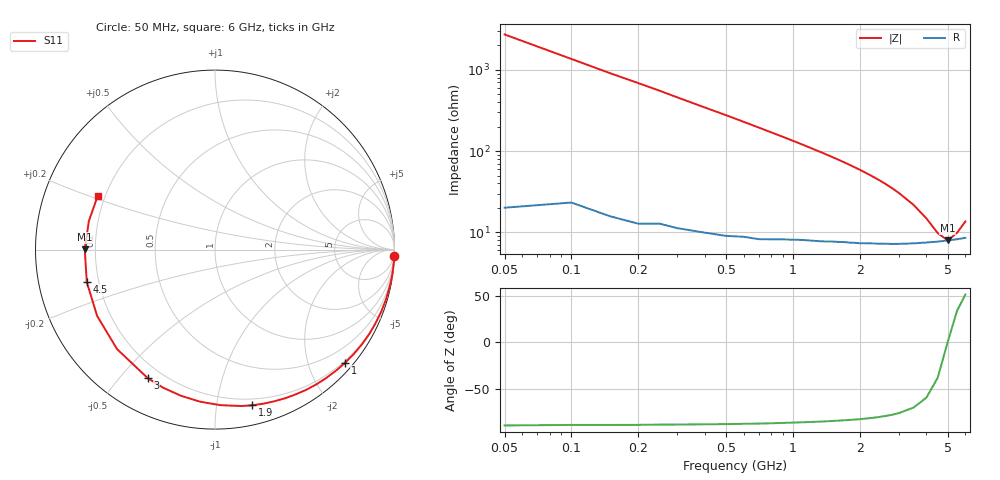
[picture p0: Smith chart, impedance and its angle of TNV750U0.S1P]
! SIEMENS Discrete & RF Semiconductors
! BAS70-07W
! Si Schottky Diode in SOT343
! VR = 0.75 V
! S-Parameters:  February  1997
# GHz  S  MA  R  50
!  f  S11
! GHz  MAG  ANG
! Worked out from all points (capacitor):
!   34 points, 50 MHz to 6 GHz, reference 50 ohm
!   read as one part to ground: C = 1.17 pF near 50 MHz
!   lowest |Z| = 7.95 ohm at 5 GHz (marker M1)
!   series resonance near 4.993 GHz, so ESL is about 870 pH
!   S11 on the Smith chart (normalised r, x): 50 MHz: 0, -55; 1 GHz: 0.16, -2.67; 1.9 GHz: 0.15, -1.26; 3 GHz: 0.14, -0.60; 4.5 GHz: 0.15, -0.12; 6 GHz: 0.17, +0.21
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0.05  0.9997 -2.1
0.2  0.9973 -8.3
0.3  0.9948 -12.4
0.4  0.9919 -16.5
0.5  0.9886 -20.5
0.6  0.9841 -24.6
0.7  0.9799 -28.7
0.8  0.9741 -32.8
0.9  0.9678 -36.8
1  0.961 -40.9
1.2  0.9467 -49.0
1.3  0.9395 -53.0
1.4  0.9321 -56.9
1.6  0.9157 -64.8
1.8  0.8997 -72.7
1.9  0.8914 -76.6
2  0.884 -80.4
2.2  0.867 -88.1
2.4  0.8513 -95.7
2.6  0.8361 -103.1
2.8  0.8222 -110.4
3  0.8083 -117.6
3.5  0.7779 -134.6
4  0.7537 -150.6
4.5  0.7369 -165.8
5  0.7258 179.8
5.5  0.7204 167.2
6  0.7188 155.4
